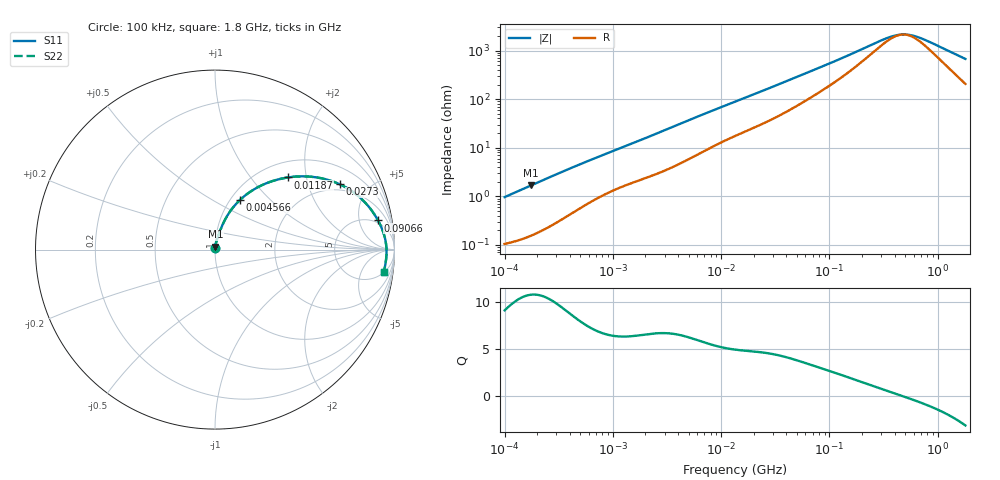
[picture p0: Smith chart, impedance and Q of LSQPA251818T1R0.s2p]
! LSQPA251818T1R0  S-PARAMETER MODEL  ( General Type )
! Model Generated by TAIYO YUDEN Corporation (http://www.ty-top.com)
! Version 4.0
! TAIYO YUDEN Control No. 160907NG19SB-FKC
! Copyright(c) 2007 TAIYO YUDEN CO.,LTD. All Rights Reserved.
! Product Description (link to TY-COMPAS)
! https://ds.yuden.co.jp/TYCOMPAS/or/detail?pn=LSQPA251818T1R0M&u=M
! Products Name : Inductors
! Characteristics :
!  Inductance : 1.0 uH , SRF(min) : 100 MHz , DC Resistance(max) : 0.104 Ohm
!  Rated Current : Saturation :1000 mA , Temp Rise : 1200 mA (40 degC)
!  Case Size : 2.5 x 1.8 / 0.098 x 0.071 [mm/inch] , Thickness : 1.8 / 0.071 [mm/inch]
!  (Conditions: Temperature = 25 degC , DC Bias Current/Voltage = 0A / 0V)
! External Node Assignments :
!  1  o---GGG---o  2
! GND o---------o GND
! Frequency Range : 0.1MHz  -  1800MHz  [ 402 STEP ]
# MHz S RI R 50
! Freq[MHz].  S11 Real  S11 Imag  S21 Real  S21 Imag  S12 Real  S12 Imag  S22 Real  S22 Imag
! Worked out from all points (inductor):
!   401 points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, 100 kHz to 1.8 GHz, reference 50 ohm
!   read as one part in series: L = 1.52 uH near 105 kHz
!   highest Q = 10.8 at 175.7 kHz (marker M1), where L = 1.52 uH
!   self-resonance near 477.8 MHz
!   S11 on the Smith chart (normalised r, x): 100 kHz: 1.00, +0.02; 4.566 MHz: 1.10, +0.67; 11.87 MHz: 1.31, +1.56; 27.3 MHz: 1.71, +3.24; 90.66 MHz: 4, +9; 1.8 GHz: 5, -13
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0.1  0.00114 0.00957  0.9989 -0.00957  0.9989 -0.00957  0.00114 0.00957
0.175662  0.00183 0.0167  0.9982 -0.0167  0.9982 -0.0167  0.00183 0.0167
0.516129  0.00809 0.0463  0.9919 -0.0463  0.9919 -0.0463  0.00809 0.0463
1.277529  0.0265 0.1001  0.9735 -0.1001  0.9735 -0.1001  0.0265 0.1001
2.66389  0.0656 0.1842  0.9344 -0.1842  0.9344 -0.1842  0.0656 0.1842
4.566214  0.1367 0.2742  0.8633 -0.2742  0.8633 -0.2742  0.1367 0.2742
7.096489  0.2395 0.3481  0.7605 -0.3481  0.7605 -0.3481  0.2395 0.3481
11.86985  0.4047 0.4018  0.5953 -0.4018  0.5953 -0.4018  0.4047 0.4018
13.41641  0.4483 0.4067  0.5517 -0.4067  0.5517 -0.4067  0.4483 0.4067
18.90474  0.5725 0.4012  0.4275 -0.4012  0.4275 -0.4012  0.5725 0.4012
27.2988  0.6958 0.3635  0.3042 -0.3635  0.3042 -0.3635  0.6958 0.3635
42.42587  0.8084 0.2895  0.1916 -0.2895  0.1916 -0.2895  0.8084 0.2895
69.24595  0.8835 0.2033  0.1165 -0.2033  0.1165 -0.2033  0.8835 0.2033
90.65972  0.9085 0.1622  0.0915 -0.1622  0.0915 -0.1622  0.9085 0.1622
167.2511  0.9406 0.0875  0.0594 -0.0875  0.0594 -0.0875  0.9406 0.0875
357.3983  0.9541 0.0215  0.0459 -0.0215  0.0459 -0.0215  0.9541 0.0215
413.9822  0.955 0.0105  0.045 -0.0105  0.045 -0.0105  0.955 0.0105
467.921  0.9554 0.00152  0.0446 -0.00152  0.0446 -0.00152  0.9554 0.00152
528.8877  0.9556 -0.00749  0.0444 0.00749  0.0444 0.00749  0.9556 -0.00749
612.6219  0.9555 -0.0185  0.0445 0.0185  0.0445 0.0185  0.9555 -0.0185
802.0705  0.9545 -0.0399  0.0455 0.0399  0.0455 0.0399  0.9545 -0.0399
1800  0.9393 -0.1271  0.0607 0.1271  0.0607 0.1271  0.9393 -0.1271
